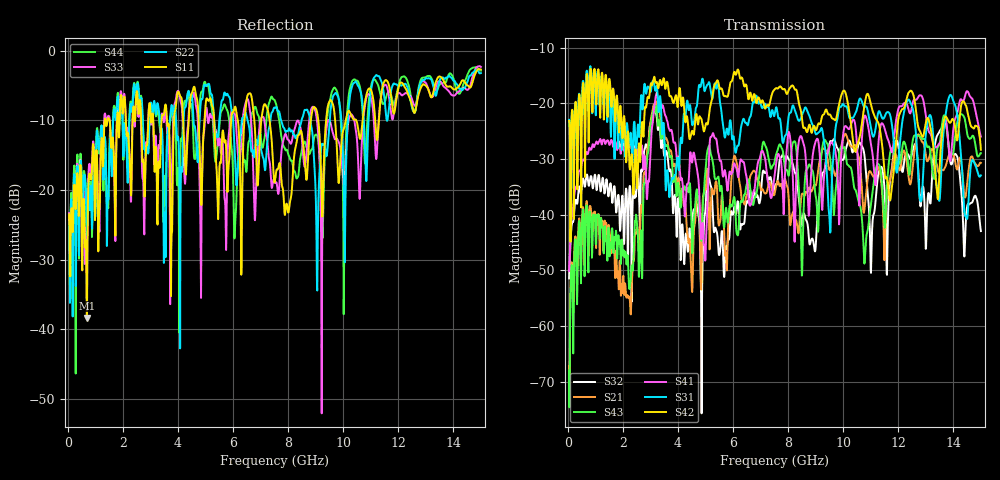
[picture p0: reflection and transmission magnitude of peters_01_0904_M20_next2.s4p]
# MHZ S RI R 50.00
! FREQ  S11  S12  S13  S14
!  S21  S22  S23  S24
!  S31  S32  S33  S34
!  S41  S42  S43  S44
!  REAL  IMAG  REAL  IMAG  REAL  IMAG  REAL  IMAG
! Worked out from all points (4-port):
!   1496 points, 50 MHz to 15 GHz, reference 50 ohm
!   strongest paths, dB at 50 MHz, 3.79 GHz, 7.53 GHz, 11.27 GHz, 15 GHz:
!     S42: -23.2, -19.3, -17.4, -23.5, -28.4
!     S31: -23.0, -33.4, -21.5, -21.7, -33.0
!     S41: -50.2, -25.3, -32.0, -27.9, -26.0
!     S43: -68.0, -30.8, -30.0, -30.9, -29.0
!     S21: -67.1, -29.9, -35.8, -31.5, -30.7
!     S32: -51.5, -35.3, -34.7, -32.9, -43.0
!   lowest |S11| = -38.4 dB at 690 MHz (marker M1), VSWR 1.02, Z = 50.5 - j1.12 ohm
!   |S11| at or under -10 dB: start of sweep to 1.339 GHz; 5.317 GHz to 5.935 GHz (617.5 MHz wide, 11 % of centre); 7.327 GHz to 8.826 GHz (1.499 GHz wide, 18.6 % of centre)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
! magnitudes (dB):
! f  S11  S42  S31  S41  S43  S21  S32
! 50 MHz  -23.5  -23.2  -23.0  -50.2  -68.0  -67.1  -51.5
! 690 MHz  -38.4  -14.8  -14.1  -28.8  -38.4  -37.6  -32.8
! 2.25 GHz  -15.6  -31.8  -26.9  -26.4  -52.9  -55.2  -34.9
! 3.17 GHz  -15.9  -16.0  -17.6  -19.8  -21.6  -20.3  -21.3
! 4.49 GHz  -6.2  -25.3  -22.7  -30.1  -41.1  -51.5  -45.2
! 9.22 GHz  -21.0  -22.6  -24.5  -37.6  -28.7  -28.7  -33.3
! 15 GHz  -2.7  -28.4  -33.0  -26.0  -29.0  -30.7  -43.0
